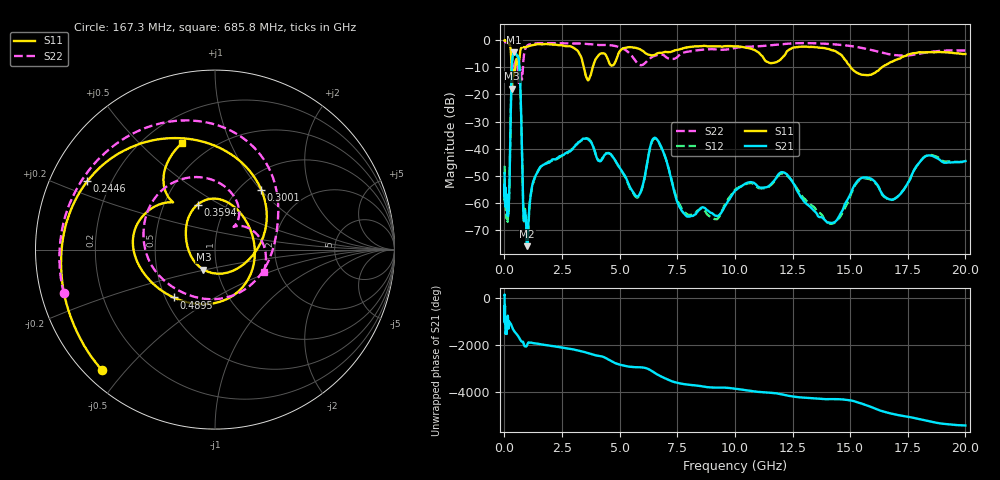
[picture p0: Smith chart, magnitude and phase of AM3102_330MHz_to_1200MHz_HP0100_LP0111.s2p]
! Date/Time: Tue, Sep 11, 2018 5:13 PM
! Network Analyzer: Agilent Technologies E8362B Rev: A.07.50.63
! Sweep from 0.010 to 20.000 GHz, 1601 Points, Sweep Type: LOG
! Power Supply: 4.949 V, 0.001 A
# Hz S DB R 50
!freq MagS11 AngS11 MagS21 AngS21 MagS12 AngS12 MagS22 AngS22
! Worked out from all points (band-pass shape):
!   1601 points, 10 MHz to 20 GHz, reference 50 ohm
!   highest |S21| = -4.39 dB at 430.5 MHz (marker M1); lowest = -76.1 dB at 993.4 MHz (marker M2)
!   |S21| within 3 dB of the highest: 338.5 MHz to 629.1 MHz (290.6 MHz wide, 60.1 % of centre)
!   lowest |S11| = -17.8 dB at 330 MHz (marker M3), VSWR 1.30, Z = 42.9 - j9.71 ohm
!   |S11| at or under -10 dB: 307.6 MHz to 474.6 MHz (166.9 MHz wide, 42.7 % of centre); 3.445 GHz to 3.829 GHz (384 MHz wide, 10.6 % of centre); 15.03 GHz to 16.37 GHz (1.346 GHz wide, 8.57 % of centre)
!   |S22| runs from -15.7 to -0.2 dB; largest |S21 - S12| = 0.01
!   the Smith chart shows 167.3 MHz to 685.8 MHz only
!   S11 on the Smith chart (normalised r, x): 167.3 MHz: 0.05, -0.43; 244.6 MHz: 0.11, +0.25; 300.1 MHz: 1.24, +1.01; 359.4 MHz: 0.73, +0.40; 489.5 MHz: 0.55, -0.34; 685.8 MHz: 0.35, +0.67
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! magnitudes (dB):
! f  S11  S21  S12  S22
! 10 MHz  0.0  -49.1  -46.4  -0.2
! 35.55 MHz  0.0  -59.7  -57.8  -0.4
! 126.4 MHz  -0.4  -63.9  -62.9  -1.0
! 167.3 MHz  -0.7  -62.6  -62.1  -1.1
! 244.6 MHz  -1.9  -42.3  -42.0  -1.8
! 300.1 MHz  -7.5  -16.8  -16.9  -3.9
! 330 MHz  -17.8  -8.5  -8.6  -7.7
! 359.4 MHz  -11.4  -5.9  -6.0  -10.6
! 430.5 MHz  -12.7  -4.4  -4.4  -9.6
! 447.2 MHz  -11.6  -4.4  -4.5  -8.8
! 489.5 MHz  -9.1  -4.7  -4.8  -7.5
! 685.8 MHz  -4.2  -15.8  -15.8  -10.5
! 829.3 MHz  -2.5  -64.7  -65.0  -7.0
! 993.4 MHz  -2.3  -76.1  -74.9  -1.9
! 1.59 GHz  -1.5  -46.6  -46.6  -1.0
! 3.582 GHz  -14.2  -36.3  -36.2  -1.3
! 5.652 GHz  -2.6  -57.0  -57.4  -7.1
! 6.58 GHz  -5.0  -36.2  -36.5  -5.5
! 7.92 GHz  -2.6  -65.1  -64.3  -4.2
! 12.09 GHz  -6.1  -48.8  -49.2  -1.4
! 14.07 GHz  -3.2  -67.4  -67.5  -1.3
! 20 GHz  -5.0  -44.7  -45.1  -3.7
